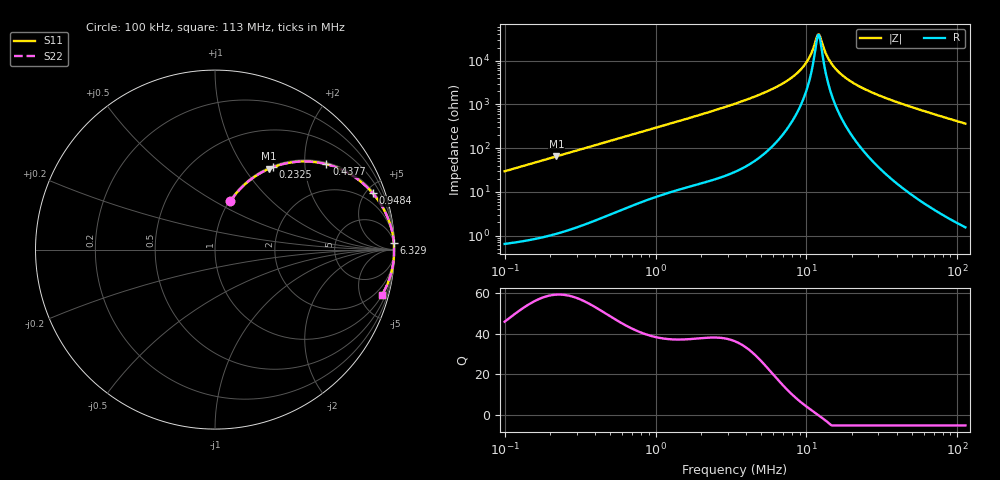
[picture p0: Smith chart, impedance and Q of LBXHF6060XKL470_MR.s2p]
! LBXHF6060XKL470_MR  S-PARAMETER MODEL  ( General Type )
! Model Generated by TAIYO YUDEN Corporation (http://www.ty-top.com)
! Version 1.0
! TAIYO YUDEN Control No. 220210
! Copyright(c) 2022 TAIYO YUDEN CO.,LTD. All Rights Reserved.
! Product Description (link to TY-COMPAS)
! https://ds.yuden.co.jp/TYCOMPAS/or/detail?pn=LBXHF6060XKL470MMR&u=M
! Products Name : Inductors
! Characteristics :
!  Inductance : 47 uH , SRF(min) : 8.5 MHz , DC Resistance(max) : 0.32 Ohm
!  Rated Current : Saturation :1000 mA , Temp Rise : 1270 mA
!  Case Size : 6.0 x 6.0 / 0.236 x 0.236 [mm/inch] , Thickness : 3 / 0.118 [mm/inch]
!  (Conditions: Temperature = 25 degC , DC Bias Current/Voltage = 0A / 0V)
! External Node Assignments :
!  1  o---GGG---o  2
! GND o---------o GND
! Frequency Range : 0.1MHz  -  113.020708MHz  [ 402 STEP ]
# MHz S RI R 50
! Freq[MHz].  S11 Real  S11 Imag  S21 Real  S21 Imag  S12 Real  S12 Imag  S22 Real  S22 Imag
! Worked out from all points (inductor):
!   401 points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, 100 kHz to 113 MHz, reference 50 ohm
!   read as one part in series: L = 47 uH near 103.6 kHz
!   highest Q = 59.1 at 220.5 kHz (marker M1), where L = 46.9 uH
!   self-resonance near 11.92 MHz
!   S11 on the Smith chart (normalised r, x): 100 kHz: 1.01, +0.59; 232.5 kHz: 1.02, +1.37; 437.7 kHz: 1.05, +2.57; 948.4 kHz: 1.14, +5.54; 6.329 MHz: 4, +50; 113 MHz: 1.03, -7.30
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0.1  0.0855 0.2689  0.9145 -0.2689  0.9145 -0.2689  0.0855 0.2689
0.149815  0.1682 0.365  0.8318 -0.365  0.8318 -0.365  0.1682 0.365
0.220536  0.3003 0.45  0.6997 -0.45  0.6997 -0.45  0.3003 0.45
0.232476  0.3225 0.459  0.6775 -0.459  0.6775 -0.459  0.3225 0.459
0.324641  0.4779 0.4907  0.5221 -0.4907  0.5221 -0.4907  0.4779 0.4907
0.437687  0.6211 0.4754  0.3789 -0.4754  0.3789 -0.4754  0.6211 0.4754
0.948442  0.8785 0.3141  0.1215 -0.3141  0.1215 -0.3141  0.8785 0.3141
1.053921  0.8983 0.2894  0.1017 -0.2894  0.1017 -0.2894  0.8983 0.2894
3.421463  0.9887 0.0927  0.0113 -0.0927  0.0113 -0.0927  0.9887 0.0927
6.32941  0.9963 0.0394  0.00373 -0.0394  0.00373 -0.0394  0.9963 0.0394
7.679361  0.997 0.0264  0.003 -0.0264  0.003 -0.0264  0.997 0.0264
8.995414  0.9973 0.0167  0.00269 -0.0167  0.00269 -0.0167  0.9973 0.0167
9.995822  0.9974 0.0105  0.00257 -0.0105  0.00257 -0.0105  0.9974 0.0105
10.91398  0.9975 0.0055  0.00251 -0.0055  0.00251 -0.0055  0.9975 0.0055
11.70886  0.9975 0.00151  0.00246 -0.00151  0.00246 -0.00151  0.9975 0.00151
12.12775  0.9976 -0.000483  0.00245 0.000483  0.00245 0.000483  0.9976 -0.000483
12.34279  0.9976 -0.00148  0.00244 0.00148  0.00244 0.00148  0.9976 -0.00148
14.20615  0.9976 -0.00953  0.0024 0.00953  0.0024 0.00953  0.9976 -0.00953
16.93579  0.9975 -0.02  0.00247 0.02  0.00247 0.02  0.9975 -0.02
22.83308  0.9968 -0.0396  0.00323 0.0396  0.00323 0.0396  0.9968 -0.0396
35.43129  0.993 -0.0757  0.00704 0.0757  0.00704 0.0757  0.993 -0.0757
113.0207  0.9292 -0.2543  0.0708 0.2543  0.0708 0.2543  0.9292 -0.2543
